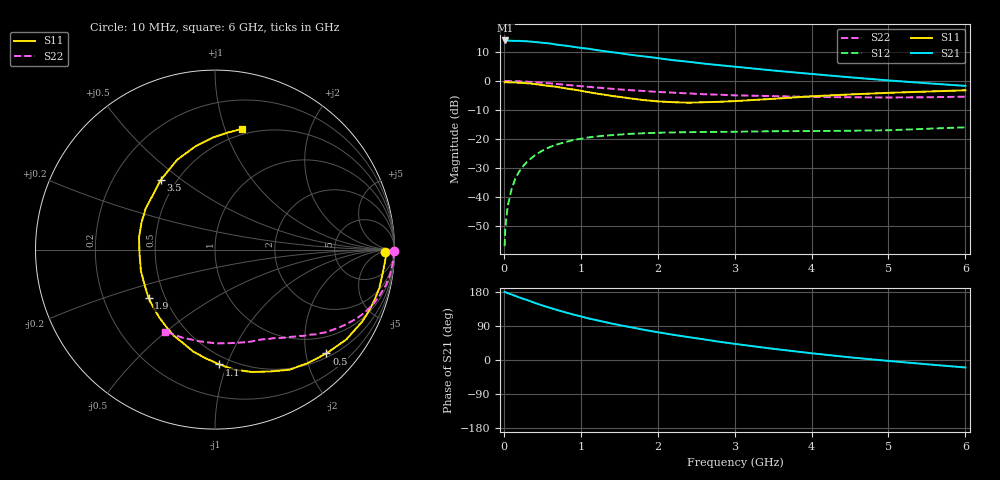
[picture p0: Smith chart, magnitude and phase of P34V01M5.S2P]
! SIEMENS Small Signal Semiconductors
! BFP181
! Si NPN RF Bipolar Junction Transistor in SOT143
! VCE = 4 V  IC = 1.5 mA
! Common Emitter S-Parameters:  March  1996
# GHz  S  MA  R  50
!  f  S11  S21  S12  S22
! GHz  MAG  ANG  MAG  ANG  MAG  ANG  MAG  ANG
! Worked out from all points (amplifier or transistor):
!   36 points, 10 MHz to 6 GHz, reference 50 ohm
!   highest |S21| = 14.0 dB at 20 MHz (marker M1)
!   |S21| within 3 dB of that: start of sweep to 1.133 GHz
!   unconditionally stable (mu >= 1): 2.756 GHz to end of sweep
!   at 250 MHz: K = 0.10, MSG = 21.6 dB, |S12| = -29.5 dB
!   at 1.4 GHz: K = 0.57, MSG = 14.3 dB, |S12| = -18.7 dB
!   at 6 GHz: K = 1.19, MAG = 4.5 dB, |S12| = -16.0 dB
!   S11 on the Smith chart (normalised r, x): 10 MHz: 34, -10; 500 MHz: 0.58, -2.42; 1.1 GHz: 0.43, -0.94; 1.9 GHz: 0.41, -0.28; 3.5 GHz: 0.41, +0.42; 6 GHz: 0.45, +1.15
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0.01  0.9474 -0.9  5.002 179.4  0.0014 97.0  0.9978 -0.4
0.02  0.9539 -1.6  5.008 179.0  0.003 94.3  0.9958 -0.8
0.05  0.9494 -4.1  4.983 176.3  0.0069 87.9  0.9959 -2.1
0.1  0.9427 -8.8  4.944 172.8  0.0134 84.9  0.9937 -4.0
0.15  0.9402 -13.2  4.92 169.0  0.0207 81.2  0.989 -6.0
0.25  0.9229 -21.9  4.882 161.5  0.0335 76.4  0.9791 -10.0
0.3  0.9131 -26.1  4.845 158.5  0.04 73.4  0.9711 -11.9
0.4  0.8865 -34.4  4.718 150.9  0.0517 68.5  0.953 -15.5
0.5  0.8487 -43.0  4.569 143.9  0.0625 63.3  0.9327 -19.0
0.6  0.8158 -50.9  4.44 137.6  0.0724 58.9  0.909 -22.2
0.8  0.745 -65.7  4.071 125.7  0.0882 50.5  0.8598 -27.7
1.1  0.64 -87.9  3.603 109.8  0.1058 40.5  0.7912 -34.5
1.3  0.5813 -102.0  3.279 100.8  0.1133 35.0  0.7511 -38.3
1.5  0.5315 -115.6  3.034 92.2  0.1184 30.6  0.7144 -41.5
1.9  0.4575 -144.0  2.586 76.9  0.1259 23.6  0.6594 -47.3
2.2  0.4299 -163.7  2.287 66.6  0.1292 19.7  0.628 -51.3
2.8  0.4365 159.4  1.873 48.2  0.132 14.3  0.579 -59.5
3.5  0.4914 128.1  1.516 29.6  0.1354 10.4  0.5478 -70.0
4  0.5433 112.8  1.322 17.8  0.1364 8.8  0.5302 -79.1
4.5  0.5848 100.9  1.156 7.0  0.1381 7.4  0.5228 -89.2
5.5  0.6556 83.8  0.913 -11.3  0.1493 7.9  0.5229 -110.2
6  0.6899 77.3  0.822 -19.7  0.1583 6.9  0.5348 -121.2
